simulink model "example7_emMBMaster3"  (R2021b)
settings: Solver=FixedStepAuto  StartTime=0  StopTime=inf  FixedStep=0.5  RelTol=1e-3  EnableMultiTasking=on
undefined symbols (not defined in the file or in its folder): based, classic, Coils, Discretes, dsPic33, InputsReg, MCC, Microchip, PIC24, Read
libraries: emMBMastedLib x10, embeddedCreatorLib x8, emMBSlaveLib x1

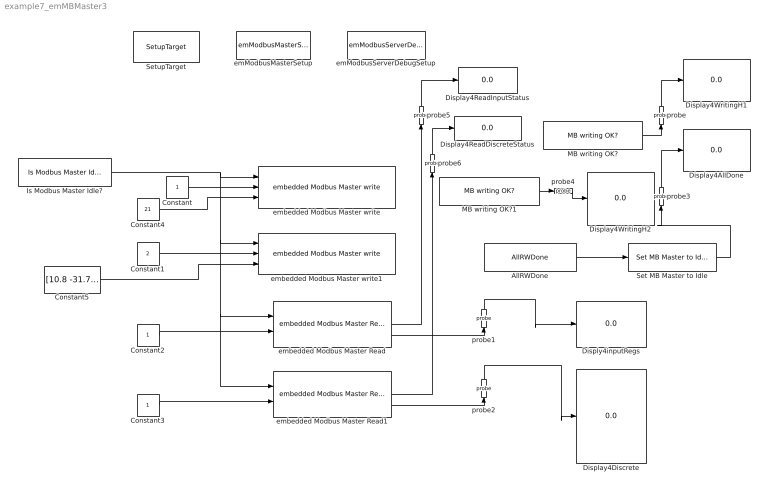
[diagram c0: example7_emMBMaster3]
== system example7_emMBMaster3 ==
  AllRWDone : emMBMastedLib/AllRWDone  c_sampleTime=-1
  Constant : Constant  OutDataTypeStr=uint16
  Constant1 : Constant  Value=2  OutDataTypeStr=uint16
  Constant2 : Constant  OutDataTypeStr=uint16
  Constant3 : Constant  OutDataTypeStr=uint16
  Constant4 : Constant  Value=21  OutDataTypeStr=uint16
  Constant5 : Constant  Value=[10.8 -31.77]  OutDataTypeStr=single
  Display4AllDone : Display
  Display4Discrete : Display
  Display4ReadDiscreteStatus : Display
  Display4ReadInputStatus : Display
  Display4WritingH1 : Display
  Display4WritingH2 : Display
  Disply4inputRegs : Display
  Is Modbus Master Idle? : emMBMastedLib/Is Modbus Master Idle?  Tag=isMB_Idle  c_sampleTime=-1
  MB writing OK? : emMBMastedLib/MB writing OK?  c_writeNo=1  c_sampleTime=-1
  MB writing OK?1 : emMBMastedLib/MB writing OK?  c_writeNo=2  c_sampleTime=-1
  Set MB Master to Idle : emMBMastedLib/Set MB Master to Idle  Tag=setMB2Idle
  SetupTarget : embeddedCreatorLib/SetupTarget  Tag=SetupTarget  Priority=0  c_platform=Microchip PIC24/dsPic33 based on MCC classic  c_debug=on
  emModbusMasterSetup : emMBMastedLib/emModbusMasterSetup  Tag=emModbusMasterSetup  c_uartNo=1  c_baudrate=19200  c_forceLongerSpace=on  c_writeServerID="[2  4 7 ]"  c_writeCMD1Type=Single-Write-holding  c_writeCMD2Type=Multiple-Write-holdings  c_writeCMD3Type=Multiple-Write-coils  c_writeCMD4Type=Single-Write-holding  c_writeCMD5Type=Single-Write-holding  c_writeCMD6Type=Single-Write-holding  c_writeCMD7Type=Single-Write-holding  c_writeCMD8Type=Single-Write-holding  c_writeCMD9Type=Single-Write-holding  c_writeCMD10Type=Single-Write-holding  c_writeCMD11Type=Single-Write-holding  c_writeCMD12Type=Single-Write-holding  c_writeCMD13Type=Single-Write-holding  c_writeCMD14Type=Single-Write-holding  c_writeCMD15Type=Single-Write-holding  c_writeRegMAXQTY=[1 8 45]  c_readCMD1Type=Read-InputsReg  c_readCMD2Type=Read-Discretes  c_readCMD3Type=Read-Coils  c_readCMD4Type=Read-Discretes  c_readCMD5Type=Read-InputsReg  c_readCMD6Type=Read-InputsReg  c_readCMD7Type=Read-InputsReg  c_readCMD8Type=Read-InputsReg  c_readCMD9Type=Read-InputsReg  c_readCMD10Type=Read-InputsReg  c_readCMD11Type=Read-InputsReg  c_readCMD12Type=Read-InputsReg  c_readCMD13Type=Read-InputsReg  c_readCMD14Type=Read-InputsReg  c_readCMD15Type=Read-InputsReg  c_readCMD16Type=Read-InputsReg  c_readRegMAXQTY=[30 7 200 300 5 6 7 8 9 10 11 12 13 14 15]  c_MaxTry=10  c_Timeout=800  c_Name_method=By phycical port name and bit number  c_PortName=B  c_BitNo=2  c_txEnable485="\"LATBbits.LATB2\""  c_TxEnable485Polarity=on
  emModbusServerDebugSetup : emMBSlaveLib/emModbusServerDebugSetup  Tag=emModbusSlaveSetup  c_objID=0  c_uartNo=2  c_baudrate=19200  c_serverID=1  c_baudrate4PC=19200  c_forceLongerSpace=on  c_holdingRegsQTY=1000  c_minHoldingAddr=789  c_inputRegsQTY=200  c_minInputRegAddr=20  c_coilRegsQTY=300  c_minCoilAddr=30  c_discreteRegsQTY=400  c_minDiscreteAddr=40  c_enableDebug=on  c_breakpointMaxQTY=100  c_probeMaxWordQTY=200  c_emWaitQTY=0  g_COMPortNo=COM5  c_Name_method=By physical port name and bit number  c_PortName=B  c_BitNo=11  c_TxEnable485="\"LATBbits.LATB11\""  c_TxEnable485Polarity=on
  embedded Modbus Master Read : emMBMastedLib/embedded Modbus Master Read  Tag=ModbusMasterReading  c_SeverID=1  c_readNo=1  c_dataType=Unsigned 32 bits int  c_dataQTY=2  c_endian=Big-endian
  embedded Modbus Master Read1 : emMBMastedLib/embedded Modbus Master Read  Tag=ModbusMasterReading  c_SeverID=2  c_readNo=2  c_dataType=Logical boolean  c_dataQTY=7  c_endian=Big-endian
  embedded Modbus Master write : emMBMastedLib/embedded Modbus Master write  Tag=ModbusMasterWriting  c_SeverID=[1 2]  c_writeNo=1  c_endian=Big-endian
  embedded Modbus Master write1 : emMBMastedLib/embedded Modbus Master write  Tag=ModbusMasterWriting  c_SeverID=[3 4]  c_writeNo=2  c_endian=Big-endian
  probe : embeddedCreatorLib/probe  Tag=emProbe  c_ObjID=5  c_serverID=1  c_UartNo=2  c_StartAddr=19  c_ConstantDataSource=off
  probe1 : embeddedCreatorLib/probe  Tag=emProbe  c_ObjID=3  c_serverID=1  c_UartNo=2  c_StartAddr=14  c_ConstantDataSource=off
  probe2 : embeddedCreatorLib/probe  Tag=emProbe  c_ObjID=0  c_serverID=1  c_UartNo=2  c_StartAddr=2  c_ConstantDataSource=off
  probe3 : embeddedCreatorLib/probe  Tag=emProbe  c_ObjID=6  c_serverID=1  c_UartNo=2  c_StartAddr=21  c_ConstantDataSource=off
  probe4 : embeddedCreatorLib/probe  Tag=emProbe  c_ObjID=2  c_serverID=1  c_UartNo=2  c_StartAddr=10  c_ConstantDataSource=off
  probe5 : embeddedCreatorLib/probe  Tag=emProbe  c_ObjID=4  c_serverID=1  c_UartNo=2  c_StartAddr=18  c_ConstantDataSource=off
  probe6 : embeddedCreatorLib/probe  Tag=emProbe  c_ObjID=1  c_serverID=1  c_UartNo=2  c_StartAddr=9  c_ConstantDataSource=off
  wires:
  Is Modbus Master Idle?/1 -> embedded Modbus Master write/1, embedded Modbus Master write1/1, embedded Modbus Master Read1/1, embedded Modbus Master Read/1
  Constant/1 -> embedded Modbus Master write/2
  AllRWDone/1 -> Set MB Master to Idle/1
  Constant4/1 -> embedded Modbus Master write/3
  Constant5/1 -> embedded Modbus Master write1/3
  Constant1/1 -> embedded Modbus Master write1/2
  Constant2/1 -> embedded Modbus Master Read/2
  Constant3/1 -> embedded Modbus Master Read1/2
  MB writing OK?/1 -> probe/1
  probe/1 -> Display4WritingH1/1
  embedded Modbus Master Read/3 -> probe1/1
  probe1/1 -> Disply4inputRegs/1
  embedded Modbus Master Read1/3 -> probe2/1
  probe2/1 -> Display4Discrete/1
  Set MB Master to Idle/1 -> probe3/1
  probe3/1 -> Display4AllDone/1
  MB writing OK?1/1 -> probe4/1
  probe4/1 -> Display4WritingH2/1
  embedded Modbus Master Read/2 -> probe5/1
  probe5/1 -> Display4ReadInputStatus/1
  embedded Modbus Master Read1/2 -> probe6/1
  probe6/1 -> Display4ReadDiscreteStatus/1
